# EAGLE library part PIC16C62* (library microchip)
MICROCONTROLLER EPROM/ROM-based
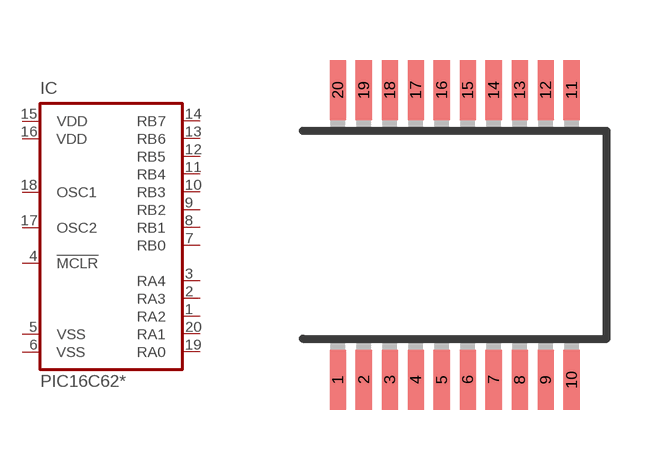
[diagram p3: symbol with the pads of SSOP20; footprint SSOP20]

Designator prefix IC

## PIC16C620SS (MF: MICROCHIP; MPN: PIC16C620A-40/SS; OC_FARNELL: unknown; OC_NEWARK: 92C4421), PIC16C621SS (MF: MICROCHIP; MPN: PIC16C621-20I/SS; OC_FARNELL: unknown; OC_NEWARK: 23C3915), PIC16C622SS (MF: MICROCHIP; MPN: PIC16C622A-04/SS; OC_FARNELL: unknown; OC_NEWARK: 23C3980)  [SSOP20]
1  RA2
2  RA3
3  RA4
4  !MCLR  in
5  VSS  pwr
6  VSS  pwr
7  RB0
8  RB1
9  RB2
10  RB3
11  RB4
12  RB5
13  RB6
14  RB7
15  VDD  pwr
16  VDD  pwr
17  OSC2  out
18  OSC1  in
19  RA0
20  RA1

## Footprint SSOP20 (pad centres in mm)
Shrink Small Outline Package package type SS
smd 0.4 x 1.5: 1 -2.925,-3.625; 2 -2.275,-3.625; 3 -1.625,-3.625; 4 -0.975,-3.625; 5 -0.325,-3.625; 6 0.325,-3.625; 7 0.975,-3.625; 8 1.625,-3.625; 9 2.275,-3.625; 10 2.925,-3.625; 11 2.925,3.625; 12 2.275,3.625; 13 1.625,3.625; 14 0.975,3.625; 15 0.325,3.625; 16 -0.325,3.625; 17 -0.975,3.625; 18 -1.625,3.625; 19 -2.275,3.625; 20 -2.925,3.625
